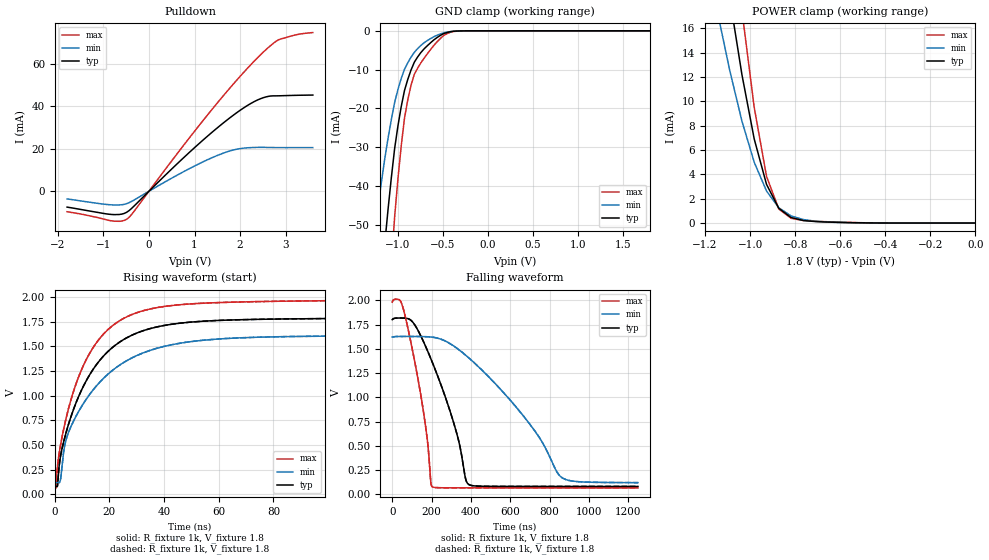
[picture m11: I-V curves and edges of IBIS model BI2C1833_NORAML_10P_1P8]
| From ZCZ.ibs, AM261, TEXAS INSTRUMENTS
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[Model]   BI2C1833_NORAML_10P_1P8
Model_type   I/O_open_drain
Polarity   Non-Inverting
Enable   Active-Low
Vinl =  0.54
Vinh =  1.26
Cref =  400pF
Rref =  528
Vref =  1.8V
Vmeas =  0.9
C_comp   2.858406p   2.529817p   3.16381p
|[Input load] normal
|[Output drive] i2c standard
|[supplytol] 10
|[temp] ind
[Model Spec]
Vinl   0.54   0.486   0.594
Vinh   1.26   1.134   1.386
[Temperature Range]   25   125   -40
[Voltage Range]   1.8   1.62   1.98
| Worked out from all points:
|   slope of the pulldown table from 0 to 0.27 V, typ, clamps not added: 47.3 ohm
|   GND clamp passes 1 mA (typ) near -0.51 V on its own axis
|   POWER clamp passes 1 mA (typ) near -0.86 V on its own axis
|   rising waveform, R_fixture 1k, V_fixture 1.8: 20-80 % time 17.4ns typ, 21ns min, 15.1ns max; typ from 0.08 V to 1.8 V
|   rising waveform, R_fixture 1k, V_fixture 1.8: 20-80 % time 17.4ns typ, 21ns min, 15.1ns max; typ from 0.08 V to 1.8 V
|   falling waveform, R_fixture 1k, V_fixture 1.8: 20-80 % time 167ns typ, 358ns min, 92.4ns max; typ from 1.8 V to 0.081 V
|   falling waveform, R_fixture 1k, V_fixture 1.8: 20-80 % time 167ns typ, 358ns min, 92.4ns max; typ from 1.8 V to 0.081 V
| Nom Voltages:
|   VDD=1.1001, VDDS=1.8, VDDS18=1.8, ESD_BIASFET=0, VSS=0, VSSS=0
| Min Voltages:
|   VDD=0.99, VDDS=1.62, VDDS18=1.62, ESD_BIASFET=0, VSS=0, VSSS=0
| Max Voltages:
|   VDD=1.21, VDDS=1.98, VDDS18=1.98, ESD_BIASFET=0, VSS=0, VSSS=0
[POWER_clamp]
|   voltage   I(typ)   I(min)   I(max)
-1.8V     125.6mA    90.89mA    174.1mA
-1.127V   23.23mA    15.78mA    33.46mA
-1.073V   16.42mA    11.17mA    23.65mA
-1.055V   14.31mA    9.772mA    20.55mA
-1.036V   12.19mA    8.372mA    17.45mA
-1.018V   10.43mA    7.246mA    14.8mA
-981.8mV  6.903mA    4.996mA    9.497mA
-927.3mV  3.179mA    2.632mA    3.84mA
-872.7mV  1.209mA    1.257mA    1.153mA
-818.2mV  452.5uA    585uA      387.7uA
-654.5mV  79.53uA    79.04uA    104.6uA
0V        23.06nA    140.3nA    354.4nA
[Pulldown]
|   voltage   I(typ)   I(min)   I(max)
-1.8V     -7.503mA   -3.655mA   -9.689mA
-818.2mV  -10.98mA   -6.45mA    -14mA
-600mV    -10.81mA   -6.386mA   -14.08mA
-490.9mV  -9.941mA   -5.873mA   -13.24mA
-327.3mV  -6.99mA    -4.156mA   -9.47mA
1.255V    25.37mA    14.53mA    35.12mA
1.745V    34.08mA    18.77mA    47.85mA
2.127V    39.93mA    20.4mA     57.12mA
2.509V    44.07mA    20.67mA    65.52mA
2.836V    44.97mA    20.56mA    71.29mA
3.218V    45.2mA     20.56mA    73.69mA
3.6V      45.33mA    20.57mA    74.8mA
[GND_clamp]
|   voltage   I(typ)   I(min)   I(max)
-1.8V     -251.3mA   -159.1mA   -395.2mA
-1.255V   -84.32mA   -51.1mA    -135.4mA
-1.145V   -54.62mA   -32.82mA   -87.84mA
-1.109V   -45.84mA   -27.58mA   -73.48mA
-1.073V   -37.72mA   -22.78mA   -60.15mA
-1.036V   -30.26mA   -18.42mA   -47.83mA
-963.6mV  -19.52mA   -12.26mA   -29.65mA
-927.3mV  -15.37mA   -9.897mA   -22.49mA
-854.5mV  -10.08mA   -6.778mA   -14.01mA
-636.4mV  -3.04mA    -1.976mA   -4.779mA
-345.5mV  -61.12uA   -61.97uA   -91.06uA
1.8V      23.06nA    171.3nA    312.3nA
[Ramp]
| variable   typ   min   max
dV/dt_f  1.0421385/0.16906483u 0.90494077/0.36005027u  1.1678122/94.773502n
dV/dt_r 71.604308m/0.85098861n 62.323663m/1.7221033n 70.734353m/0.6449258n
R_load = 1k
[Rising Waveform]
R_fixture = 1k
V_fixture = 1.8
V_fixture_min = 1.62
V_fixture_max = 1.98
|   time   V(typ)   V(min)   V(max)
0s        79.89mV    118.4mV    66.28mV
428.7ps   79.89mV    118.4mV    66.28mV
958.7ps   84.73mV    118.4mV    275.1mV
1.959ns   363.7mV    135.1mV    475.9mV
3.653ns   577.5mV    498.4mV    712.5mV
6.175ns   808.5mV    703.6mV    983.7mV
15.93ns   1.34V      1.122V     1.563V
29.61ns   1.631V     1.402V     1.838V
52.01ns   1.752V     1.556V     1.935V
1.25us    1.8V       1.62V      1.98V
[Rising Waveform]
R_fixture = 1k
V_fixture = 1.8
V_fixture_min = 1.62
V_fixture_max = 1.98
|   time   V(typ)   V(min)   V(max)
0s        79.89mV    118.4mV    66.28mV
428.7ps   79.89mV    118.4mV    66.28mV
958.7ps   84.73mV    118.4mV    275.1mV
1.959ns   363.7mV    135.1mV    475.9mV
3.653ns   577.5mV    498.4mV    712.5mV
6.175ns   808.5mV    703.6mV    983.7mV
15.93ns   1.34V      1.122V     1.563V
29.61ns   1.631V     1.402V     1.838V
52.01ns   1.752V     1.556V     1.935V
1.25us    1.8V       1.62V      1.98V
[Falling Waveform]
R_fixture = 1k
V_fixture = 1.8
V_fixture_min = 1.62
V_fixture_max = 1.98
|   time   V(typ)   V(min)   V(max)
0s        1.801V     1.621V     1.981V
43.5ns    1.818V     1.628V     1.987V
80.76ns   1.811V     1.628V     1.704V
160.7ns   1.567V     1.626V     828.5mV
204.1ns   1.36V      1.62V      77.1mV
311.7ns   743.4mV    1.531V     66.21mV
390.9ns   98.95mV    1.404V     66.04mV
689.6ns   80.72mV    750mV      65.97mV
863.6ns   80.68mV    171.3mV    65.97mV
1.25us    80.67mV    119.8mV    65.97mV
[Falling Waveform]
R_fixture = 1k
V_fixture = 1.8
V_fixture_min = 1.62
V_fixture_max = 1.98
|   time   V(typ)   V(min)   V(max)
0s        1.801V     1.621V     1.981V
43.5ns    1.818V     1.628V     1.987V
80.76ns   1.811V     1.628V     1.704V
160.7ns   1.567V     1.626V     828.5mV
204.1ns   1.36V      1.62V      77.1mV
311.7ns   743.4mV    1.531V     66.21mV
390.9ns   98.95mV    1.404V     66.04mV
689.6ns   80.72mV    750mV      65.97mV
863.6ns   80.68mV    171.3mV    65.97mV
1.25us    80.67mV    119.8mV    65.97mV
